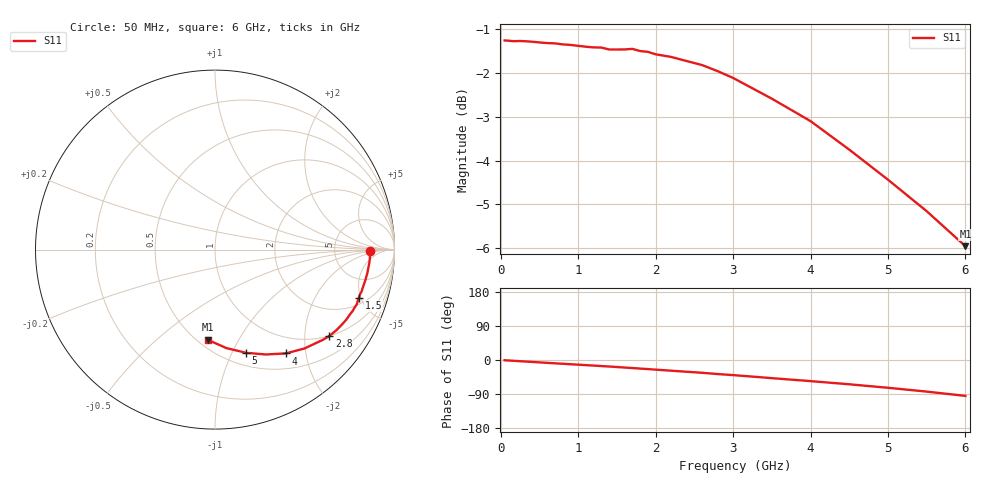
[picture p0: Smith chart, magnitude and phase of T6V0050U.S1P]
! SIEMENS Discrete & RF Semiconductors
! BAT62
! Si Schottky Diode in SOT143
! IF = 0.05 mA
! S-Parameters:  February  1997
# GHz  S  MA  R  50
!  f  S11
! GHz  MAG  ANG
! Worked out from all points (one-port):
!   34 points, 50 MHz to 6 GHz, reference 50 ohm
!   lowest |S11| = -6.0 dB at 6 GHz (marker M1), VSWR 3.03, Z = 27.9 - j37.6 ohm
!   |S11| at or under -10 dB: nowhere
!   S11 on the Smith chart (normalised r, x): 50 MHz: 14, -1; 1.5 GHz: 2.57, -4.82; 2.8 GHz: 1.00, -2.65; 4 GHz: 0.73, -1.65; 5 GHz: 0.63, -1.13; 6 GHz: 0.56, -0.75
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0.05  0.8655 -0.6
0.2  0.864 -2.6
0.4  0.8628 -5.0
0.7  0.8589 -8.8
0.8  0.8566 -9.9
0.9  0.8555 -11.2
1  0.8534 -12.3
1.1  0.8514 -13.6
1.2  0.8499 -14.7
1.3  0.8495 -16.0
1.4  0.8452 -17.2
1.5  0.8452 -18.5
1.6  0.8453 -19.9
1.7  0.8466 -21.2
1.8  0.8417 -22.7
1.9  0.84 -23.9
2  0.8346 -25.5
2.2  0.8288 -28.2
2.4  0.8199 -31.0
2.6  0.8113 -33.7
2.8  0.7985 -37.1
3  0.7843 -39.8
3.5  0.7427 -47.9
4  0.7001 -55.7
4.5  0.6496 -64.1
5  0.6002 -73.3
5.5  0.5524 -83.4
6  0.5039 -94.7
